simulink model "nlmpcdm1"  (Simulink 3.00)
settings: Solver=ode45  SolverMode=SingleTasking  StartTime=0.0  StopTime=4  MaxStep=0.2  RelTol=1e-3  AbsTol=1e-6
PreLoadFcn:
  | demo1dat
libraries: nlmpclib x1

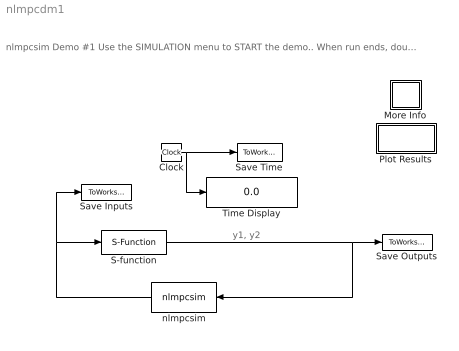
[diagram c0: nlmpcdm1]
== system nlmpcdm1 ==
  note: y1, y2
  note: nlmpcsim Demo #1 Use the SIMULATION menu to START the demo.. When run ends, double click on PLOT RESULTS. (Double click on the "?" for more info)
  Clock : Clock
  More Info : Subsystem
  Plot Results : Subsystem
  S-function : S-Function  FunctionName=mpcplant  PortCounts=[]  SFunctionModules=''
  Save Inputs : ToWorkspace  VariableName=u  SampleTime=0
  Save Outputs : ToWorkspace  VariableName=y  SampleTime=0
  Save Time : ToWorkspace  VariableName=t  SampleTime=0
  Time Display : Display
  nlmpcsim : nlmpclib/nlmpcsim  Orientation=left
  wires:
  S-function/1 -> Save Outputs/1, nlmpcsim/1
  nlmpcsim/1 -> S-function/1, Save Inputs/1
  Clock/1 -> Save Time/1, Time Display/1

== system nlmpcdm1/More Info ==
  note: After the simulation ends, double-click on "Plot Results". Inputs and outputs will be plotted in a figure window using the MPC Tools "ploteach" command.
  note: Use the Simulation menu to Start the simulation.
  note: This demonstration shows how masked variables are specified for nlmpcsim. See the manual for details.

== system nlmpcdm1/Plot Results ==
